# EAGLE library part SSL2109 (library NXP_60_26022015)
Compact non-dimmable LED driver IC The SSL2109T is a high-voltage Integrated Circuit (IC) for driving LED lamps in general lighting applications. The main benefits of this IC include: • Small Printed-Circuit Board (PCB) footprint and compact solution • High efficiency (up to 95 %) for non-dimmable high power factor solutions • High power factor >0.9 (application dependent) • Ease of integration and many protection features • Low electronic Bill Of Material (BOM) • Highly flexible IC for use in buck, buck/boost and flyback modes • Single inductor used for non-isolated configurations because of internal demagnetization detection and dV/dt supply The IC is supplementary to the SSL21081/SSL21083 series but without an internal switch. The IC has been designed to start up directly from the HV supply by an internal high-voltage current source. Thereafter, the dV/dt supply is used with capacitive coupling from the drain, or any other auxiliary supply. This functionality provides full flexibility in the application design. An internal clamp limits the supply voltage. The IC provides accurate output current control to within 5 % LED current accuracy. The IC can be operated using Pulse-Width Modulation (PWM) current regulation and has many protection features including easy LED temperature feedback. AAL Eindhoven MK
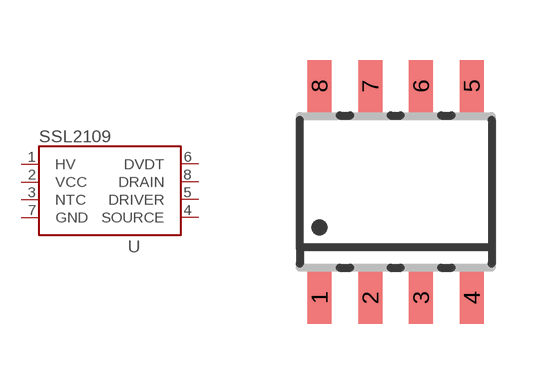
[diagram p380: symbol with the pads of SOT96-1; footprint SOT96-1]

Designator prefix U

## SSL2109T, SSL2109AT  [SOT96-1]
1  HV  pwr
2  VCC  pwr
3  NTC  pas
4  SOURCE  pas
5  DRIVER  pas
6  DVDT  pas
7  GND  pwr
8  DRAIN  pas

## Footprint SOT96-1 (pad centres in mm)
SOT96-1 SO8: plastic small outline package; 8 leads; body width 3.9 mm JEDEC: MS-012 IEC: 076E03
smd 0.6 x 1.3: 1 -1.905,-2.65; 2 -0.635,-2.65; 3 0.635,-2.65; 4 1.905,-2.65; 5 1.905,2.65; 6 0.635,2.65; 7 -0.635,2.65; 8 -1.905,2.65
